DATA_BLOCK DB 21
TITLE =
AUTHOR : Gersch
FAMILY : Modul
VERSION : 0.0

 FB 20
BEGIN
   pi_fu_adr_in := P#P  0.0;
   pi_fu_adr_out := P#P  0.0;
   db_sys_sd := DB 1;
   bii_1_bwg_pf := FALSE;
   bii_1_reset := FALSE;
   bii_1_frg := FALSE;
   bii_1_ref_auto_asf := FALSE;
   bii_1_ref_hand_asf := FALSE;
   bii_1_tip_neg := FALSE;
   bii_1_tip_pos := FALSE;
   bii_1_mot_stop := FALSE;
   bii_1_mot_fkt_asf := FALSE;
   bii_1_mot_fkt_start := FALSE;
   bii_1_mot_fkt_start_pf := FALSE;
   bii_1_mot_strom_nenn := FALSE;
   bii_do_01_anst := FALSE;
   bii_do_02_anst := FALSE;
   bii_do_03_anst := FALSE;
   bii_do_04_anst := FALSE;
   by_fkt_mod := B#16#0;
   bii_1_vfs_prio := FALSE;
   ii_vfs_nr := 0;
   rei_sw_v_tip := 0.000000e+000;
   rei_sw_v_reg := 0.000000e+000;
   rei_sw_vr := 0.000000e+000;
   rei_sw_i := 0.000000e+000;
   rei_sw_pos := 0.000000e+000;
   rei_sw_ruck := 0.000000e+000;
   rei_sw_zt_pos := 0.000000e+000;
   rei_ref_auto_io_ev := 0.000000e+000;
   rei_ref_hand_swv := 0.000000e+000;
   rei_ref_hand_zt_pos := 0.000000e+000;
   rei_ref_hand_rel_pos := 0.000000e+000;
   rei_sm_zt_max_kom := 0.000000e+000;
   dii_ztw_zyklus := L#0;
   dii_sf_cod := L#0;
   bio_1_bm := FALSE;
   bio_1_sm := FALSE;
   byo_bmnr := B#16#0;
   byo_smnr := B#16#0;
   byo_sm_info_cmd := B#16#0;
   byo_sm_info_mnr := B#16#0;
   reo_sm_info_data := 0.000000e+000;
   bio_1_kom_io := FALSE;
   bio_1_ref_io_fu := FALSE;
   bio_1_ref_io_fb := FALSE;
   bio_1_ref_frg_bwg := FALSE;
   bio_1_prog_akt := FALSE;
   bio_1_bremse_fest := FALSE;
   bio_1_bewegung_vhr := FALSE;
   bio_1_mot_blockiert := FALSE;
   bio_1_fkt_io := FALSE;
   bio_1_fkt_nio := FALSE;
   bio_di_01_status := FALSE;
   bio_di_02_status := FALSE;
   bio_di_03_status := FALSE;
   bio_di_04_status := FALSE;
   io_fkt_vfs_nr := 0;
   reo_fkt_sw_i := 0.000000e+000;
   reo_fkt_sw_pos := 0.000000e+000;
   reo_iw_v := 0.000000e+000;
   reo_iw_i := 0.000000e+000;
   reo_iw_pos := 0.000000e+000;
   out.bm := FALSE;
   out.sm := FALSE;
   out.bmnr := B#16#0;
   out.smnr := B#16#0;
   out.sm_info_cmd := B#16#0;
   out.sm_info_mnr := B#16#0;
   out.sm_info_data := 0.000000e+000;
   out.kom_io := FALSE;
   out.ref_io_fu := FALSE;
   out.ref_io_fb := FALSE;
   out.ref_frg_bwg := FALSE;
   out.prog_akt := FALSE;
   out.bremse_akt := FALSE;
   out.bewegung_vhr := FALSE;
   out.mot_blockiert := FALSE;
   out.fkt_io := FALSE;
   out.fkt_nio := FALSE;
   out.fkt_nio_pf := FALSE;
   out.di_01_status := FALSE;
   out.di_02_status := FALSE;
   out.di_03_status := FALSE;
   out.di_04_status := FALSE;
   out.fkt_vfs_nr := 0;
   out.fkt_sw_i := 0.000000e+000;
   out.fkt_sw_pos := 0.000000e+000;
   out.iw_v := 0.000000e+000;
   out.iw_i := 0.000000e+000;
   out.iw_pos := 0.000000e+000;
   sd.kom_zhw_delta := FALSE;
   sd.not_stop_pf := FALSE;
   sd.not_stop_pfs := FALSE;
   sd.quit_pf := FALSE;
   sd.quit_pfs := FALSE;
   sd.ref_akt := FALSE;
   sd.ref_auto_asf_pf := FALSE;
   sd.ref_auto_asf_pfs := FALSE;
   sd.ref_hand_asf_pf := FALSE;
   sd.ref_hand_asf_pfs := FALSE;
   sd.mot_fkt_start_pf := FALSE;
   sd.mot_fkt_start_pfs := FALSE;
   sd.mot_fkt_asf_zsp := FALSE;
   sd.mot_fkt_asf_pf := FALSE;
   sd.mot_fkt_asf_pfs := FALSE;
   sd.mot_fkt_start_pf_pf := FALSE;
   sd.mot_fkt_start_pf_asf := FALSE;
   sd.mot_fkt_start := FALSE;
   sd.mot_ini_io := FALSE;
   sd.bd_tip := FALSE;
   sd.bd_tip_neg := FALSE;
   sd.tip_neg_pf := FALSE;
   sd.tip_neg_pfs_zsp := FALSE;
   sd.bd_tip_pos := FALSE;
   sd.tip_pos_pf := FALSE;
   sd.tip_pos_pfs_zsp := FALSE;
   sd.tip_akt := FALSE;
   sd.frg_mot := FALSE;
   sd.mot_stop := FALSE;
   sd.frg_baa := FALSE;
   sd.vfs_prio_asf := FALSE;
   sd.vfs_prio_zsp := FALSE;
   sd.vfs_prio_pf := FALSE;
   sd.reg_swv_i := FALSE;
   sd.reg_pos_io_zsp := FALSE;
   sd.sts07_pose_pf := FALSE;
   sd.frg_baa_pf := FALSE;
   sd.frg_baa_pfs := FALSE;
   sd.lb_adr_erm := FALSE;
   sd.zykl_spl_akt := FALSE;
   sd.fkt_mod_delta := FALSE;
   sd.fkt_mod_zsp := B#16#0;
   sd.lb_adr_adr_zsp00 := 0;
   sd.lb_adr_adr_zsp01 := 0;
   sd.lb_adr_adr_zsp02 := 0;
   sd.czw_zsp := B#16#0;
   sd.fkt_mod_asf := B#16#0;
   sd.fkt_spl := 0;
   sd.fkt_spl_zsp := 0;
   sd.fkt_spl_zhw := 0;
   sd.zykl_spl := 0;
   sd.sw_v_asf := L#0;
   sd.sw_v_vrg := 0.000000e+000;
   sd.sw_v_reg_zsp := 0.000000e+000;
   sd.sw_vr_zsp := 0.000000e+000;
   sd.sw_i_zsp := 0.000000e+000;
   sd.sw_pos_vrg := 0.000000e+000;
   sd.sw_pos_zsp := 0.000000e+000;
   sd.sw_ruck_zsp := 0.000000e+000;
   sd.sw_zt_pos_vrg := 0.000000e+000;
   sd.sw_zt_pos_zsp := 0.000000e+000;
   sd.reg_vfs_nr_zsp := 0;
   sd.reg_sw_i_zsp := 0.000000e+000;
   sd.reg_sw_pos_zsp := 0.000000e+000;
   sd.vrg_sw_v_reg := 0.000000e+000;
   sd.vrg_sw_vr := 0.000000e+000;
   sd.vrg_sw_i := 0.000000e+000;
   sd.vrg_sw_pos := 0.000000e+000;
   sd.vrg_sw_ruck := 0.000000e+000;
   sd.vrg_sw_zt_pos := 0.000000e+000;
   sd.sys_fb_zhw := L#0;
   sd.ref_auto_io_ev := L#0;
   sd.zts01 := FALSE;
   sd.zts02 := FALSE;
   sd.ztw01 := L#0;
   sd.ztvg01_kom_max := L#0;
   sd.ztvg01_kom_max_spl := L#0;
   sd.ztw02 := L#0;
   sd.ztw03 := L#0;
   sd.ztw04 := L#0;
   sd.ztw05 := L#0;
   sd.ztw06_ref := L#0;
   sd.ztw07_ref_io := L#0;
   sd.in_sw_v_reg_zsp := 0.000000e+000;
   sd.in_sw_vr_zsp := 0.000000e+000;
   sd.in_sw_ruck_zsp := 0.000000e+000;
   sd.in_sw_i_zsp := 0.000000e+000;
   sd.in_sw_zt_pos_zsp := 0.000000e+000;
   cmd.commando_io := FALSE;
   cmd.commando_neu := FALSE;
   cmd.commando_wechsel := FALSE;
   cmd.cmd_frg_bwg := FALSE;
   cmd.cmd_bwg_asf := FALSE;
   cmd.ack_io := FALSE;
   cmd.ack_asf := FALSE;
   cmd.ref_baa_io := FALSE;
   cmd.ref_auto_asf := FALSE;
   cmd.ref_hand_asf := FALSE;
   cmd.ref_hand_cmd_erh := FALSE;
   cmd.ref_hand_cmd_frg_jog := FALSE;
   cmd.get_info_asf := FALSE;
   cmd.get_info_pf := FALSE;
   cmd.stop_io := FALSE;
   cmd.stop_asf := FALSE;
   cmd.not_stop_io := FALSE;
   cmd.not_stop_asf := FALSE;
   cmd.get_state_io := FALSE;
   cmd.get_di_do_io := FALSE;
   cmd.get_konfig_io := FALSE;
   cmd.get_erro_info_io := FALSE;
   cmd.fkt_mod_zsp := B#16#0;
   cmd.get_konfig_nr := 0;
   mot.config.ehsys := B#16#0;
   mot.config.r002 := 0;
   mot.config.sed_min := 0.000000e+000;
   mot.config.sed_max := 0.000000e+000;
   mot.config.swv_max := 0.000000e+000;
   mot.config.swdv_max := 0.000000e+000;
   mot.config.swvr_max := 0.000000e+000;
   mot.config.swi_n := 0.000000e+000;
   mot.config.swi_max := 0.000000e+000;
   end := FALSE;
END_DATA_BLOCK

